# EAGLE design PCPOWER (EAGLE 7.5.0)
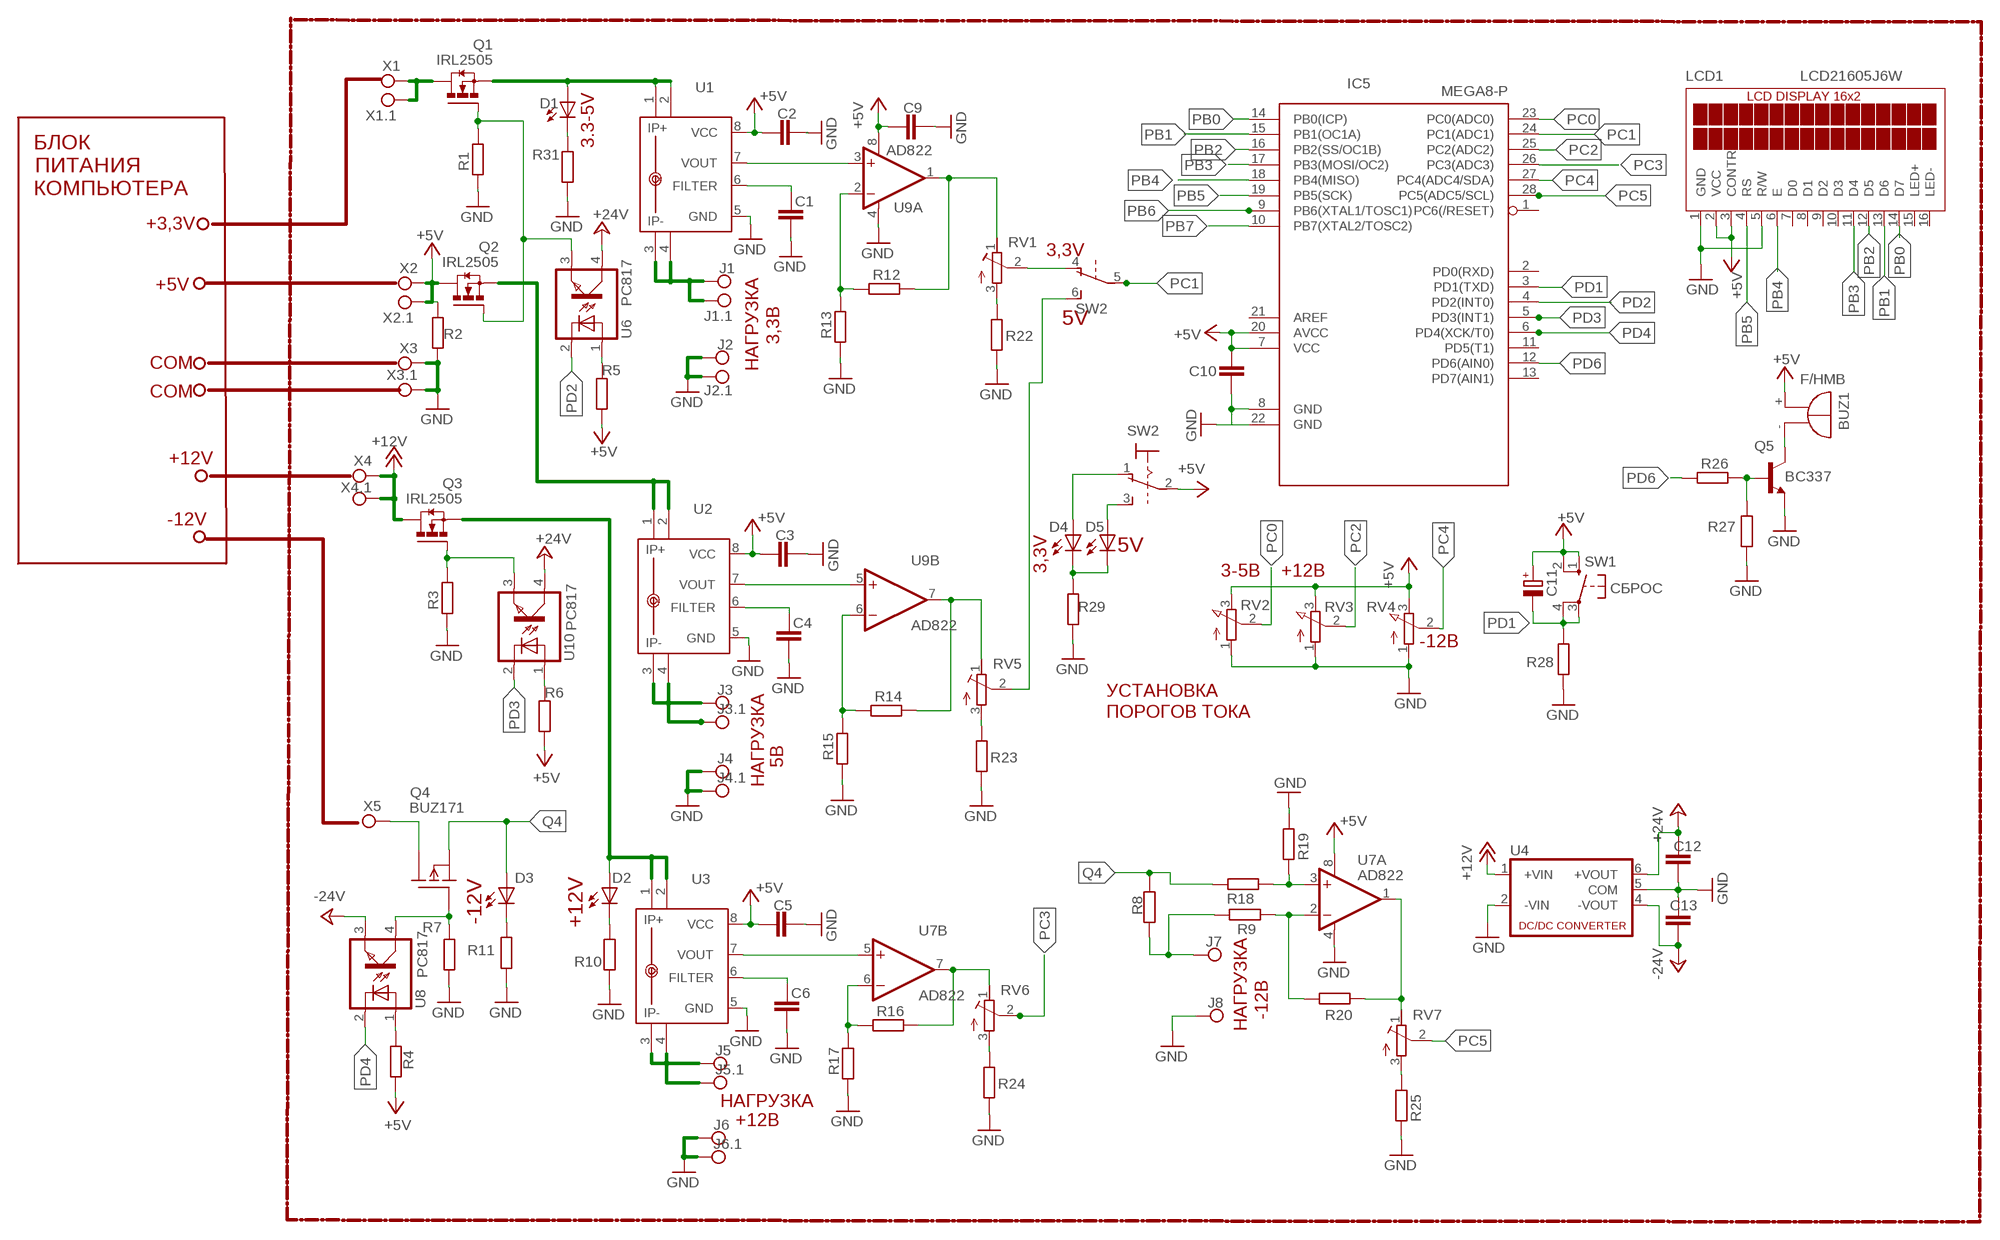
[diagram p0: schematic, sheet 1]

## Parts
BUZ1  F/HMB  [F/HMB]
C1  C-EUC1206  [C1206]
C2  C-EUC1206  [C1206]
C3  C-EUC1206  [C1206]
C4  C-EUC1206  [C1206]
C5  C-EUC1206  [C1206]
C6  C-EUC1206  [C1206]
C9  C-EUC1206  [C1206]
C10  C-EUC1206  [C1206]
C11  CPOL-EUE2-4  [E2-4]
C12  C-EUC1206  [C1206]
C13  C-EUC1206  [C1206]
D1  LED3MM  [LED3MM]
D2  LED3MM  [LED3MM]
D3  LED3MM  [LED3MM]
D4  LED3MM  [LED3MM]
D5  LED3MM  [LED3MM]
IC5  MEGA8-P  [DIL28-3]
J1  TPPAD1-20  [P1-20]
J1.1  TPPAD1-20  [P1-20]
J2  TPPAD1-20  [P1-20]
J2.1  TPPAD1-20  [P1-20]
J3  TPPAD1-20  [P1-20]
J3.1  TPPAD1-20  [P1-20]
J4  TPPAD1-20  [P1-20]
J4.1  TPPAD1-20  [P1-20]
J5  TPPAD1-20  [P1-20]
J5.1  TPPAD1-20  [P1-20]
J6  TPPAD1-20  [P1-20]
J6.1  TPPAD1-20  [P1-20]
J7  TPPAD1-20  [P1-20]
J8  TPPAD1-20  [P1-20]
LCD1  LCD21605J6W  [LCD21605J6W]
Q1  IRL2505  IRF3704L-V  [TO262-V]
Q2  IRL2505  IRF3704L-V  [TO262-V]
Q3  IRL2505  IRF3704L-V  [TO262-V]
Q4  BUZ171  [TO220]
Q5  BC337  [TO92]
R1  R-EU_R1206  [R1206]
R2  R-EU_VTA54  [VTA54]
R3  R-EU_R1206  [R1206]
R4  R-EU_R1206  [R1206]
R5  R-EU_R1206  [R1206]
R6  R-EU_R1206  [R1206]
R7  R-EU_R1206  [R1206]
R8  R-EU_0309/12  [0309/12]
R9  R-EU_R1206  [R1206]
R10  R-EU_R1206  [R1206]
R11  R-EU_R1206  [R1206]
R12  R-EU_R1206  [R1206]
R13  R-EU_R1206  [R1206]
R14  R-EU_R1206  [R1206]
R15  R-EU_R1206  [R1206]
R16  R-EU_R1206  [R1206]
R17  R-EU_R1206  [R1206]
R18  R-EU_R1206  [R1206]
R19  R-EU_R1206  [R1206]
R20  R-EU_R1206  [R1206]
R22  R-EU_R1206  [R1206]
R23  R-EU_R1206  [R1206]
R24  R-EU_R1206  [R1206]
R25  R-EU_R1206  [R1206]
R26  R-EU_R1206  [R1206]
R27  R-EU_R1206  [R1206]
R28  R-EU_R1206  [R1206]
R29  R-EU_R1206  [R1206]
R31  R-EU_R1206  [R1206]
RV1  R-TRIMM-3386-F  [R-TRIMM-3386F]
RV2  PTV09A  PV09A  [PTV09]
RV3  PTV09A  PV09A  [PTV09]
RV4  PTV09A  PV09A  [PTV09]
RV5  R-TRIMM-3386-F  [R-TRIMM-3386F]
RV6  R-TRIMM-3386-F  [R-TRIMM-3386F]
RV7  R-TRIMM-3386-F  [R-TRIMM-3386F]
SW1  SPST Push Button  10-XX  [B3F-10XX]
SW2  320-938  [320-938]
U1  ACS712ELCTR-20A-T  [SO8]
U2  ACS712ELCTR-20A-T  [SO8]
U3  ACS712ELCTR-20A-T  [SO8]
U4  NMA  [NMA]
U6  PC817  [DIL04]
U7  AD822  OPA2134P  [DIL08]
U8  PC817  [DIL04]
U9  AD822  OPA2134P  [DIL08]
U10  PC817  [DIL04]
X1  TPPAD1-20  [P1-20]
X1.1  TPPAD1-20  [P1-20]
X2  TPPAD1-20  [P1-20]
X2.1  TPPAD1-20  [P1-20]
X3  TPPAD1-20  [P1-20]
X3.1  TPPAD1-20  [P1-20]
X4  TPPAD1-20  [P1-20]
X4.1  TPPAD1-20  [P1-20]
X5  TPPAD1-20  [P1-20]

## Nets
+5V: BUZ1.+ C2.2 C3.2 C5.2 C9.2 C10.2 C11.+ IC5.7(VCC) IC5.20(AVCC) LCD1.2(VCC) LCD1.3(CONTR) Q2.2(D) R2.2 R4.2 R5.2 R6.2 RV2.3(E) RV3.3(E) RV4.3(E) SW1.1(S) SW1.2(S1) SW2.2(1:P) U1.8(VCC) U2.8(VCC) U3.8(VCC) U7.8(A:V+) U9.8(A:V+) X2.1.TP X2.TP
+12V: Q3.2(D) U4.1(+VIN) X4.1.TP X4.TP
+24V: C12.1 U4.6(+VOUT) U6.4(COL) U10.4(COL)
-24V: C13.2 U4.4(-VOUT) U8.3(EMIT)
GND: C1.2 C2.1 C3.1 C4.2 C5.1 C6.2 C9.1 C10.1 C12.2 C13.1 IC5.8(GND) IC5.22(GND) J2.1.TP J2.TP J4.1.TP J4.TP J6.1.TP J6.TP J8.TP LCD1.1(GND) LCD1.5(R/W) Q5.1(E) R1.2 R2.1 R3.2 R7.2 R10.2 R11.2 R13.2 R15.2 R17.2 R19.2 R22.2 R23.2 R24.2 R25.1 R27.2 R28.2 R29.2 R31.2 RV2.1(A) RV3.1(A) RV4.1(A) U1.5(GND) U2.5(GND) U3.5(GND) U4.2(-VIN) U4.5(COM) U7.4(A:V-) U9.4(A:V-) X3.1.TP X3.TP
N$1: R14.2 R15.1 U9.6(B:-IN)
N$2: J1.1.TP J1.TP U1.3(IP-) U1.4(IP-1)
N$3: R22.1 RV1.3(E)
N$4: Q5.2(B) R26.1 R27.1
N$5: D1.K(C) R31.1
N$6: BUZ1.- Q5.3(C)
N$7: RV1.2(S) SW2.4(B:O)
N$8: R14.1 RV5.1(A) U9.7(B:OUT)
N$9: R12.2 R13.1 U9.2(A:-IN)
N$10: R12.1 RV1.1(A) U9.1(A:OUT)
N$11: C1.1 U1.6(FILTER)
N$12: D1.A Q1.3(S) U1.1(IP+) U1.2(IP+1)
N$13: Q1.1(G) Q2.1(G) R1.1 U6.3(EMIT)
N$14: U1.7(VOUT) U9.3(A:+IN)
N$15: Q1.2(D) X1.1.TP X1.TP
N$16: R5.1 U6.1(A)
N$17: U2.7(VOUT) U9.5(B:+IN)
N$18: C4.1 U2.6(FILTER)
N$19: Q2.3(S) U2.1(IP+) U2.2(IP+1)
N$20: R23.1 RV5.3(E)
N$21: J3.1.TP J3.TP U2.3(IP-) U2.4(IP-1)
N$22: R16.2 R17.1 U7.6(B:-IN)
N$24: Q3.1(G) R3.1 U10.3(EMIT)
N$25: U3.7(VOUT) U7.5(B:+IN)
N$26: C6.1 U3.6(FILTER)
N$27: J5.1.TP J5.TP U3.3(IP-) U3.4(IP-1)
N$28: D2.K(C) R10.1
N$29: D2.A Q3.3(S) U3.1(IP+) U3.2(IP+1)
N$30: R16.1 RV6.1(A) U7.7(B:OUT)
N$31: R6.1 U10.1(A)
N$32: R24.1 RV6.3(E)
N$33: Q4.1(G) R7.1 U8.4(COL)
N$34: Q4.2(D) X5.TP
N$35: R4.1 U8.1(A)
N$36: D3.K(C) R11.1
N$37: J7.TP R8.1 R9.1
N$38: R9.2 R20.2 U7.2(A:-IN)
N$39: R18.2 R19.1 U7.3(A:+IN)
N$40: R20.1 RV7.1(A) U7.1(A:OUT)
N$41: R25.2 RV7.3(E)
N$42: D4.A SW2.1(1:O)
N$43: D5.A SW2.3(1:S)
N$44: D4.K(C) D5.K(C) R29.1
N$46: RV5.2(S) SW2.6(B:S)
PB0: IC5.14(PB0(ICP)) LCD1.14(D7)
PB1: IC5.15(PB1(OC1A)) LCD1.13(D6)
PB2: IC5.16(PB2(SS/OC1B)) LCD1.12(D5)
PB3: IC5.17(PB3(MOSI/OC2)) LCD1.11(D4)
PB4: IC5.18(PB4(MISO)) LCD1.6(E)
PB5: IC5.19(PB5(SCK)) LCD1.4(RS)
PB6: IC5.9(PB6(XTAL1/TOSC1))
PB7: IC5.10(PB7(XTAL2/TOSC2))
PC0: IC5.23(PC0(ADC0)) RV2.2(S)
PC1: IC5.24(PC1(ADC1)) SW2.5(B:P)
PC2: IC5.25(PC2(ADC2)) RV3.2(S)
PC3: IC5.26(PC3(ADC3)) RV6.2(S)
PC4: IC5.27(PC4(ADC4/SDA)) RV4.2(S)
PC5: IC5.28(PC5(ADC5/SCL)) RV7.2(S)
PD1: C11.- IC5.3(PD1(TXD)) R28.1 SW1.3(P) SW1.4(P1)
PD2: IC5.4(PD2(INT0)) U6.2(C)
PD3: IC5.5(PD3(INT1)) U10.2(C)
PD4: IC5.6(PD4(XCK/T0)) U8.2(C)
PD6: IC5.12(PD6(AIN0)) R26.2
Q4: D3.A Q4.3(S) R8.2 R18.1
Unconnected: IC5.1(PC6(/RESET)) IC5.2(PD0(RXD)) IC5.11(PD5(T1)) IC5.13(PD7(AIN1)) IC5.21(AREF) LCD1.7(D0) LCD1.8(D1) LCD1.9(D2) LCD1.10(D3) LCD1.15(LED+) LCD1.16(LED-)

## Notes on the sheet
- 3.3-5V
- БЛОК
- ПИТАНИЯ
- КОМПЬЮТЕРА
- +3,3V
- 3,3V
- +5V
- 5V
- 3,3В
- COM | НАГРУЗКА
- COM
- +12V
- -12V
- 5V
- 3-5В | +12В
- 3,3V
- СБРОС
- -12В
- УСТАНОВКА
- ПОРОГОВ ТОКА
- 5В
- НАГРУЗКА
- -12V | +12V
- -12В
- НАГРУЗКА
- НАГРУЗКА
- +12В

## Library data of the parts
BUZ1 = buzzer:F/HMB: BUZZER; OC_FARNELL: unknown; OC_NEWARK: unknown
C1-C6 C9 C10 C12 C13 = rcl:C-EU: CAPACITOR, European symbol
C11 = rcl:CPOL-EU: POLARIZED CAPACITOR, European symbol
D1-D5 = led:LED: LED
IC5 = atmel:MEGA8-P: MICROCONTROLLER 8 Kbytes FLASH, 1 kbytes SRAM, 512 bytes EEPROM, USART, 4-channel 10 bit ADC, 2-channel 8 bit ADC Pin compatible with Atmega48, ATMega88, ATMega168 Source: avr.lbr; OC_FARNELL: unknown; OC_NEWARK: unknown
J1 J1.1 J2 J2.1 J3 J3.1 J4 J4.1 J5 J5.1 J6 J6.1 J7 J8 X1 X1.1 X2 X2.1 X3 X3.1 X4 X4.1 X5 = testpad:TP: Test pad
LCD1 = display-lcd:LCD21605J6W
Q1-Q3 = transistor-power:IRF3704: SMPS MOSFET HEXFET® Power MOSFET Source: http://www.irf.com/product-info/datasheets/data/irf3704.pdf
Q4 = transistor-fet:BUZ171: P-Channel Enhancement MOSFET -50V; 7A; 0,4Ohm
Q5 = transistor:BC337: NPN TRANSISTOR
R1-R20 R22-R29 R31 = rcl:R-EU_: RESISTOR, European symbol
RV1 RV5-RV7 = rcl:R-TRIMM-3386-F
RV2-RV4 = pot:PV09A
SW1 = switch-omron:10-XX: OMRON SWITCH; MPN: B3F-1000; OC_FARNELL: 176432; OC_NEWARK: 36M3542
SW2 = switch:320-938: TOGGLE SWITCH distributor RS Components
U1-U3 = allegro:ACS712ELCTR-20A-T: Fully Integrated, Hall Effect-Based Linear Current Sensor with High Voltage Isolation and a Low-Resistance Current Conductor.
U4 = dc-dc-converter:NMA: DC-DC CONVERTER; MF: C & D TECHNOLOGIES, INC; MPN: NMA0515SC; OC_FARNELL: 1021434; OC_NEWARK: 61K3064
U6 U8 U10 = optocoupler:PC817: SHARP OPTO COUPLER; MPN: PC817X4J000F; OC_FARNELL: 9707727; OC_NEWARK: 97K7059
U7 U9 = burr-brown:OPA2134: Operational Amplifier; MF: TEXAS INSTRUMENTS; MPN: OPA2134PA; OC_FARNELL: 1097574; OC_NEWARK: 74K3897

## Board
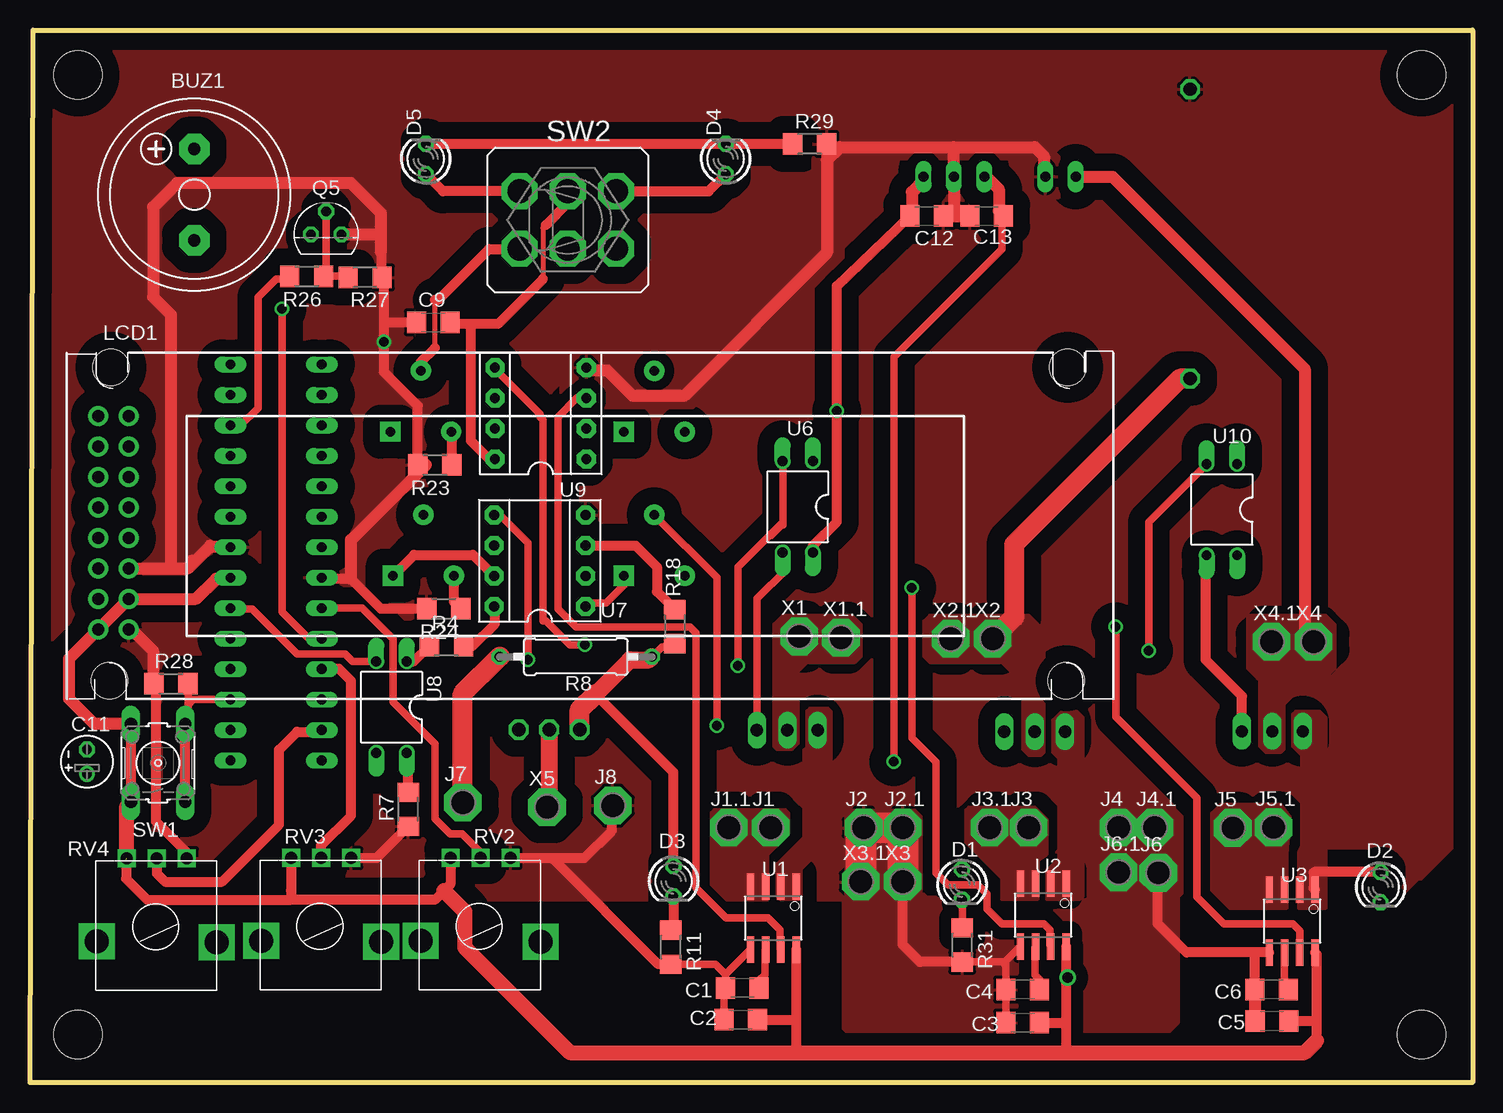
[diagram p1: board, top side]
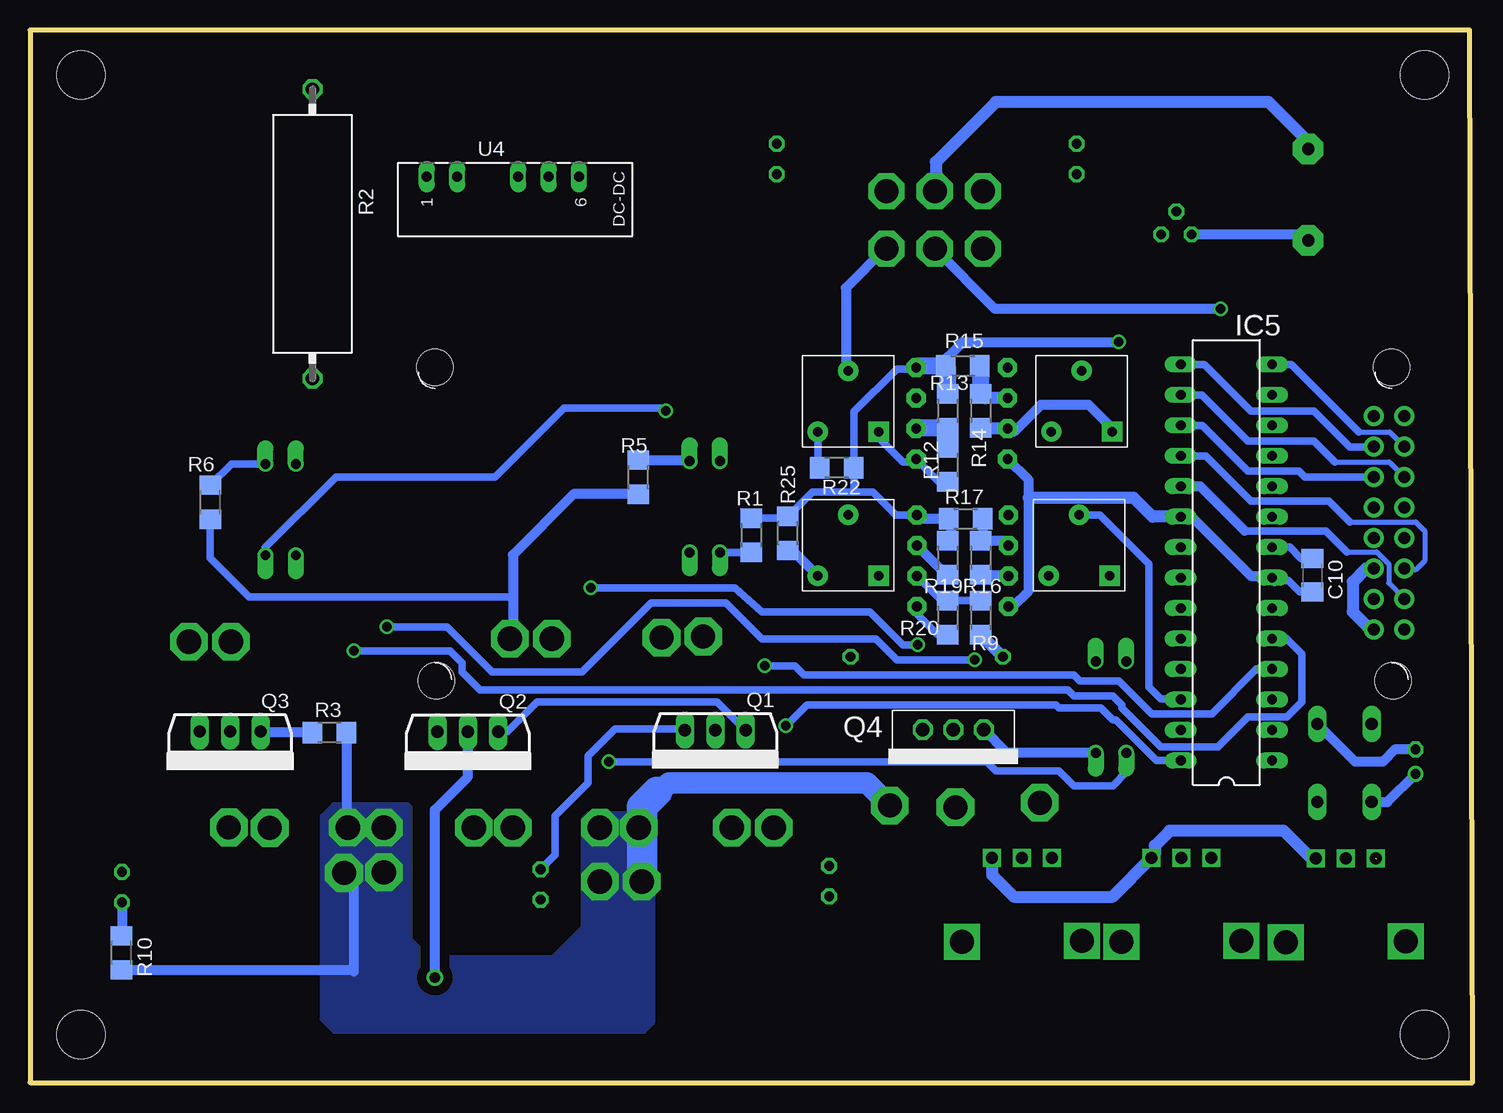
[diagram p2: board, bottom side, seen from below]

Size 120.25 x 87.75 mm. Coordinates in mm from the lower left corner, seen from the top.
Outline: 0,0 0.25,87.75 120.25,87.75 120.25,0 0,0
Copper layers (1*16): Top 0.035mm / dielectric 1.5mm / Bottom 0.035mm
Design rules "default *": minimum track width 10mil, minimum drill 24mil, track to track 5mil, track to pad 5mil, pad to pad 8mil, via to via 8mil, smd to smd 8mil, copper to edge 40mil, drill to drill 8mil, minimum pad ring 10mil, minimum via ring 8mil, stop-mask expansion 4mil, vias tented up to drill 0mil, thermal gap 10mil
Holes 4 mm at 4,84 4,4 116,4 116,84

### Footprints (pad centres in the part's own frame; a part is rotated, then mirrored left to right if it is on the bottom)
F/HMB = drill 1.016 pad 2.54 octagon: + 3.81,0; - -3.81,0
C1206 = smd 1.6 x 1.8: 1 -1.4,0; 2 1.4,0
E2-4 = drill 0.813 pad 1.27: + -1.016,0 | drill 0.813 pad 1.27 octagon: - 1.016,0
LED3MM = drill 0.813 octagon: A -1.27,0; K 1.27,0
DIL28-3 = drill 0.813 long: 1 -16.51,-3.81; 2 -13.97,-3.81; 3 -11.43,-3.81; 4 -8.89,-3.81; 5 -6.35,-3.81; 6 -3.81,-3.81; 7 -1.27,-3.81; 8 1.27,-3.81; 9 3.81,-3.81; 10 6.35,-3.81; 11 8.89,-3.81; 12 11.43,-3.81; 13 13.97,-3.81; 14 16.51,-3.81; 15 16.51,3.81; 16 13.97,3.81; 17 11.43,3.81; 18 8.89,3.81; 19 6.35,3.81; 20 3.81,3.81; 21 1.27,3.81; 22 -1.27,3.81; 23 -3.81,3.81; 24 -6.35,3.81; 25 -8.89,3.81; 26 -11.43,3.81; 27 -13.97,3.81; 28 -16.51,3.81
P1-20 = drill 2.007 pad 3.15 octagon: TP 0,0
LCD21605J6W = drill 1 pad 1.676: 1 2.47,-17.72; 2 -0.07,-17.72; 3 2.47,-15.18; 4 -0.07,-15.18; 5 2.47,-12.64; 6 -0.07,-12.64; 7 2.47,-10.1; 8 -0.07,-10.1; 9 2.47,-7.56; 10 -0.07,-7.56; 11 2.47,-5.02; 12 -0.07,-5.02; 13 2.47,-2.48; 14 -0.07,-2.48; 15 2.47,0.06; 16 -0.07,0.06 | hole 3: 0.875,-22; 1,4.125; 80.75,4.125; 80.625,-22
TO262-V = drill 1.016 long: 1 -2.54,0; 2 0,0; 3 2.54,0
TO220 = drill 1.118 octagon: 1 -2.54,0; 2 0,0; 3 2.54,0
TO92 = drill 0.813 octagon: 1 1.27,0; 2 0,1.905; 3 -1.27,0
R1206 = smd 1.6 x 1.803: 1 -1.422,0; 2 1.422,0
VTA54 = drill 1.1 octagon: 1 -12.065,0; 2 12.065,0
0309/12 = drill 0.813 octagon: 1 -6.35,0; 2 6.35,0
R-TRIMM-3386F = drill 0.8 pad 1.676 square: 1 0,0 | drill 0.8 pad 1.676: 2 5.08,2.54; 3 0,5.08
PTV09 = drill 1 square: 1 -2.5,0; 2 0,0; 3 2.5,0 | drill 2 square: P$4 -5,7; P$5 5,6.9
B3F-10XX = drill 1.016 long: 1 -3.251,2.261; 2 3.251,2.261; 3 -3.251,-2.261; 4 3.251,-2.261
320-938 = drill 2.007 octagon: 1 -2.388,4.013; 2 -2.388,0; 3 -2.388,-4.013; 4 2.388,4.013; 5 2.388,0; 6 2.388,-4.013
SO8 = smd 0.61 x 2.21: 1 0.635,-0.076; 2 1.905,-0.076; 3 3.175,-0.076; 4 4.445,-0.076; 5 4.445,5.156; 6 3.175,5.156; 7 1.905,5.156; 8 0.635,5.156
NMA = drill 0.813 long: 1 0,6.35; 2 0,3.81; 4 0,-1.27; 5 0,-3.81; 6 0,-6.35
DIL04 = drill 0.813 offset: 1 -1.27,-3.81; 2 1.27,-3.81; 3 1.27,3.81; 4 -1.27,3.81
DIL08 = drill 0.813 pad 1.6 octagon: 1 -3.81,-3.81; 2 -1.27,-3.81; 3 1.27,-3.81; 4 3.81,-3.81; 5 3.81,3.81; 6 1.27,3.81; 7 -1.27,3.81; 8 -3.81,3.81

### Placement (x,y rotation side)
BUZ1  13.7,74.02 90 top
C1  59.38,7.88 180 top
C2  59.25,5.25 0 top
C3  82.75,5 0 top
C4  82.75,7.75 180 top
C5  103.53,5.14 0 top
C6  103.5,7.75 180 top
C9  33.62,63.38 0 top
C10  13.36,42.29 270 bottom
C11  4.75,26.75 90 top
C12  74.75,72.25 0 top
C13  79.75,72.25 0 top
D1  77.69,16.51 270 top
D2  112.58,16.29 270 top
D3  53.63,16.79 270 top
D4  58,77 90 top
D5  33,77 90 top
IC5  20.51,43.36 90 bottom
J1  61.75,21.25 0 top
J1.1  58.25,21.25 0 top
J2  69.5,21.25 0 top
J2.1  72.75,21.25 0 top
J3  83.25,21.25 0 top
J3.1  80,21.25 0 top
J4  90.75,21.25 0 top
J4.1  93.75,21.25 0 top
J5  100.26,21.22 0 top
J5.1  103.67,21.27 0 top
J6  94.07,17.47 0 top
J6.1  90.75,17.52 0 top
J7  36.08,23.33 0 top
J8  48.58,23.09 0 top
LCD1  5.75,55.5 0 top
Q1  63.12,29.38 180 bottom
Q2  83.75,29.25 180 bottom
Q3  103.57,29.28 180 bottom
Q4  43.28,29.42 180 bottom
Q5  24.69,70.71 0 top
R1  60.12,45.62 90 bottom
R2  96.7,70.75 270 bottom
R3  95.29,29.17 0 bottom
R4  34.72,36.41 0 top
R5  69.53,50.47 270 bottom
R6  105.21,48.38 270 bottom
R7  31.54,22.77 270 top
R8  45.5,35.5 0 top
R9  41,38.75 90 bottom
R10  112.61,10.81 270 bottom
R11  53.42,11.29 270 top
R12  43.75,51.5 90 bottom
R13  43.75,56 90 bottom
R14  41,56 90 bottom
R15  42.5,59.75 180 bottom
R16  41,43.75 90 bottom
R17  42.25,47 180 bottom
R18  53.75,38 90 top
R19  43.75,43.75 90 bottom
R20  43.75,38.75 90 bottom
R22  53,51.25 0 bottom
R23  33.75,51.5 180 top
R24  34.5,39.5 180 top
R25  57.08,45.78 270 bottom
R26  23.06,67.21 180 top
R27  27.94,67.12 0 top
R28  11.75,33.25 180 top
R29  65,78.25 0 top
R31  77.71,11.47 270 top
RV1  49.5,54.25 90 bottom
RV2  37.55,18.72 180 top
RV3  24.27,18.72 180 top
RV4  10.57,18.69 180 top
RV5  30.04,54.26 90 bottom
RV6  30.25,42.25 90 bottom
RV7  49.5,42.25 90 bottom
SW1  10.67,26.64 90 top
SW2  44.83,71.91 270 top
U1  64.5,16.25 180 top
U2  87,16.5 180 top
U3  107.75,16 180 top
U4  80.83,75.52 90 bottom
U6  64,48 180 top
U7  42.5,43.5 90 top
U8  30.13,31.3 180 top
U9  42.57,55.79 90 top
U10  99.36,47.76 180 top
X1  64.13,37.19 0 top
X1.1  67.61,37.09 0 top
X2  80.25,37 0 top
X2.1  76.75,37 0 top
X3  72.75,16.75 0 top
X3.1  69.25,16.75 0 top
X4  107,36.75 0 top
X4.1  103.5,36.75 0 top
X5  43.1,22.95 0 top

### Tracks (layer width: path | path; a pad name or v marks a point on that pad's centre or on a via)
+5V  (via drill 0.9)  (1 unrouted)
  Top 0.406: 43,71.5 42.75,71.25 42.75,67
  Top 0.813: RV2.3 35.05,16.55 34.5,16 33.75,15.25 21.75,15.25 | 107.25,3.5 107.25,5 | 107.25,5 107.25,10.71 U3.8 | C5.2 107.11,5.14 107.25,5 | 86.36,5 U2.8 86.36,8.88 v86.5,8.75 | 86.36,5 86.36,2.63 86.5,2.5 | C3.2 86.36,5 | U1.8 63.87,5 | 63.87,5 63.87,2.62 63.75,2.5 | C2.2 63.62,5.25 63.87,5 | R4.2 36.91,36.41 38.75,38.25 38.75,39.63 U7.8 38.56,39.69 | SW1.2 SW1.1 | 8,18.62 8,17 9.75,15.25 21.75,15.25 | RV3.3 21.77,15.98 21.75,15.25 | U9.8 38.27,51.98 36.75,53.5 36.75,63.25 | 36.75,63.25 35.15,63.25 C9.2 | SW2.2 44.83,73.33 43,71.5 | 42.75,67 39,63.25 36.75,63.25
  Top 1.016: SW1.2 5.36,29.89 3.25,32 3.25,35.35 LCD1.2 LCD1.3 13.82,40.32 15.5,42 16.61,42 IC5.7
  Top 1.27: 107.25,3.5 106.25,2.5 86.5,2.5 63.75,2.5 45,2.5 36.25,11.25 36.25,14.25 34.5,16 | RV4.3 8.07,23.05 SW1.1
  Top 1.676: R2.2 95.86,58.69 82.03,44.85 82.03,38.77 X2.TP
  Bottom 0.61: R6.2 105.21,43.71 102,40.5 80.25,40.5 80,40.25 | C10.2 14.39,40.89 15.38,41.88 16.48,41.88 IC5.7
  Bottom 0.813: U7.8 38.31,39.69 37,41 37,48.75 37,50.22 U9.8 | R5.2 74.95,49.05 80,44 80,40.25 80,37.25 X2.TP | SW1.1 7.09,23.39 C11.+ | IC5.20 23.42,47.17 18.5,42.25 16.86,42.25 IC5.7 | v86.5,8.75 86.5,22.75 83.75,25.5 Q2.2
  Bottom 1.016: IC5.20 26.67,47.17 28.25,48.75 37,48.75 | 16.5,41.89 IC5.7 | BUZ1.+ 13.7,78.45 17,81.75 39.75,81.75 44.75,76.75 44.75,74.38 SW2.2
  pour Top (no thermals): 75,39 83.25,39 84.5,37.75 84.5,27.5 84.25,27.25 83.25,27.25 82.75,27.75 82.75,33.25 81,35 75,35 74.5,35.5 74.5,38.5
+12V
  Top 1.016: U4.1 90.23,75.52 106.25,59.5 106.25,36.5 X4.TP
  pour Top (no thermals): 102.5,28 102.5,33.5 101.5,34.5 101.5,39 108,39 108.75,38.25 108.75,34.5 107.75,33.5 106.5,33.5 104.5,31.5 104.5,27.75 104.25,27.5 103,27.5
+24V  (via drill 0.8)
  Top 0.813: U6.4 65.27,44.77 67.25,46.75 v67.25,56 67.25,66.4 C12.1
  Top 1.016: U4.6 74.48,75.23 73.5,74.25 73.5,72.4 C12.1
  Bottom 0.61: U10.4 100.63,44.62 94.75,50.5 81.5,50.5 75.75,56.25 67.5,56.25 v67.25,56
-24V  (via drill 0.8)
  Top 0.61: v72,26.75 72,60.5 81,69.5 81,72.1 C13.2
  Top 1.016: U4.4 79.73,75.52 80.75,74.5 80.75,72.65 C13.2
  Bottom 0.61: U8.3 28.86,25.89 30,24.75 33.25,24.75 34.5,26 39.75,26 40.5,26.75 v72,26.75
GND  (via drill 0.8)
  Top 0.61: C3.1 C4.2 81.35,9.75 | 81.35,9.75 81.35,10.14 U2.5 | R31.2 81.05,10.05 81.35,9.75 | C2.1 57.85,7.75 C1.2 57.98,9.01 | 57.98,9.01 U1.5 | R11.2 57.13,9.86 57.98,9.01
  Top 0.813: R24.2 29.25,39.5 26.75,42 24.41,42 IC5.22 | R23.2 32.33,56.42 29.5,59.25 v29.5,61.75 29.5,63.25 | 29.5,63.25 29.5,66.98 R27.2 29.25,67.23 29.25,69.25 | RV3.1 28.9,18.72 R7.2 | RV2.1 43.5,18.72 | 43.5,18.72 46.22,18.72 48.5,21 48.5,23.01 J8.TP | RV4.1 13.07,19.18 10.5,21.75 10.5,33.08 R28.2 | R11.2 52.36,9.86 43.5,18.72 | U3.5 102,10.84 | 102,10.84 96.41,10.84 94,13.25 94,17.4 J6.TP | C6.2 102.1,10.74 102,10.84 | C9.1 29.62,63.38 29.5,63.25 | R31.2 74.2,10.05 72.75,11.5 X3.TP
  Top 1.016: 26.75,42 26.75,45.25 33,51.5 R23.2 | LCD1.5 11.5,42.86 | 11.5,42.86 13.17,42.86 15,44.69 16.64,44.69 IC5.8 15.12,44.63 15,44.75 13.5,43.25 13.5,43.5 | LCD1.1 8.47,37.78 10.25,36 10.25,33.33 R28.2 | 77,78 67.5,78 66.42,76.92 R29.2 66.42,69.17 54.5,57.25 50.25,57.25 48.12,59.38 46.6,59.38 U9.4 | 77,78 83.75,78 84.5,77.25 84.5,75.66 U4.2 | 77,78 77.02,77.98 U4.5 77.02,72.48 77.25,72.25 | C12.2 77.25,72.25 | 77.25,72.25 C13.1 | 11.5,42.86 11.75,43.11 11.75,64 10.25,65.5 10.25,73 12.25,75 26.75,75 29.25,72.5 29.25,70.5 | 29.25,69.25 29.25,70.5 | Q5.1 29.04,70.71 29.25,70.5 | C6.2 102.1,5.17 C5.1
  Top 2.54: X3.TP J2.1.TP J2.TP 69.25,21 X3.1.TP
  Bottom 0.61: R1.2 57.23,47.05 R25.1 55.03,49.25 51.75,49.25 | U7.4 48.06,47.31 50,49.25 51.75,49.25 | 51.75,49.25 51.58,49.42 R22.2 51.58,55.92 48,59.5 46.48,59.5 U9.4 | C10.1 14.31,43.69 15.25,44.63 IC5.8
  Bottom 0.813: R19.2 43.5,45.42 43.5,46.75 43.67,46.92 R17.2 46,47 U7.4 | R13.2 43.75,60.5 42.5,61.75 v29.5,61.75 | R3.2 93.87,21.37 J4.1.TP | R10.2 93.39,9.39 93.25,9.25 93.25,16.65 J6.TP
  Bottom 1.016: 16.64,44.69 IC5.8 | LCD1.5 8.89,42.86 10,41.75 10,39.25 8.75,38 8.44,38 LCD1.1 | RV2.1 40.05,17.3 38.25,15.5 29.99,15.5 RV3.1 26.5,18.99 26.5,19.75 25.25,21 15.75,21 13.44,18.69 RV4.1
  Bottom 1.422: U9.4 46.23,59.75 R15.2 43.75,59.58 R13.2
  Bottom 1.778: 68,24.25 67.75,24.25 67,25 50.49,25 J8.TP
  Bottom 2.54: X3.1.TP 69.25,23 68,24.25
  pour Top (no thermals): 88.75,23 95.25,23 95.75,22.5 96,22.25 96,15.75 95.5,15.25 89.25,15.25 88.75,15.75 88.75,22.75
  pour Bottom (isolate 0.813, no thermals): 88.75,23.25 95,23.25 96,22.25 96,5.25 95,4.25 69,4.25 68.25,5 68.25,22 68.75,22.5 73.75,22.5 74.25,22 74.25,13 76.75,10.5 87,10.5 88.5,12 88.5,23
  pour Top (no thermals): 68,22.75 73.75,22.75 74.25,22.25 74.25,15.25 74,15 68.5,15 68,15.5
  pour Top (isolate 0.813): 45.25,61.75 57.25,61.75 61.75,66.25 65.25,69.75 65.25,79 66,79.75 83.25,79.75 85.75,77.25 85.75,73.75 84,73.75 83.5,74.25 83.5,76.75 83.25,77 69,77 67.75,75.75 67.75,68.75 55.25,56.25 45,56.25 44.25,57 44.25,61 45,61.75
  pour Top (isolate 1.422): 74.75,15 113.75,15 115.75,17 116,17 119.25,20.25 119.25,86.75 1.25,86.75 1.25,15.5 1.5,15.25 74.5,15.25
  pour Top (isolate 1.016): 67.75,23.25 67.75,4.5 68.25,4 94.75,4 95.75,5 95.75,22.5 95,23.25 88.75,23.25 88.5,23 88.5,15.75 88,15.25 74.75,15.5 73.75,16.5 74.25,22.25 73.25,23.25
N$1
  Bottom 1.016: U9.6 40.64,57.06 R14.2
  Bottom 1.422: R14.2 41,59.67 R15.1
N$2
  pour Top (no thermals): 61.5,15.25 61.5,19 63.25,20.75 63.25,22.5 63,22.75 57,22.75 56.75,22.5 56.75,16.5 58,15.25
N$3
  Bottom 0.61: RV1.3 54.58,51.16 R22.1
N$4
  Top 0.61: R27.1 26.43,67.21 R26.1 24.69,67.42 Q5.2
  Top 0.813: 26.39,67.25 R27.1
N$5
  Top 0.61: R31.1 77.71,15.22 D1.K
N$6
  Bottom 0.813: Q5.3 14.2,70.71 BUZ1.-
N$7
  Bottom 0.813: SW2.4 48.98,69.52 52.25,66.25 52.25,59.54 RV1.2
N$8
  Bottom 0.813: RV5.1 30.04,54.54 32,56.5 36,56.5 38.25,54.25 38.49,54.25 U9.7
  Bottom 1.016: R14.1 38.82,54.58 U9.7
N$9
  Bottom 1.422: R12.2 R13.1 46.32,54.58 U9.2
N$10
  Bottom 0.61: R12.1 44.48,50.08 U9.1 46.61,51.75 47.5,51.75 49.5,53.75 RV1.1
N$11
  Top 0.61: C1.1 60.77,8.53 61.25,9 61.25,11.02 U1.6
N$12
  Bottom 0.61: Q1.3 65.79,29.5 71.5,29.5 73.75,27.25 73.75,25 76.5,22.25 76.5,18.97 D1.A
  pour Top (no thermals): 62.25,15.5 62.25,18.25 64.5,20.5 64.5,27.75 64.75,28 64.75,31 65,31.25 66.5,31.25 66.75,31 66.75,26.5 66.25,26 66.25,19.75 64.25,17.75 64.25,15.25 62.5,15.25
N$13
  Top 0.61: Q1.1 60.59,40.34 63,42.75 63,43.92 U6.3
  Bottom 0.61: R1.1 62.72,44.2 U6.3 | Q2.1 80.5,29.25 78,31.75 62.96,31.75 Q1.1
N$14
  Top 0.61: U9.3 45.56,57.06 44,55.5 44,39.5 45.5,38 55,38 55.5,37.5 55.5,16.25 58,13.75 61.5,13.75 62.5,12.75 62.5,11.19 U1.7
N$15
  pour Top (no thermals): 62,28 62,38.25 62.75,39 68.5,39 69.25,38.25 69.25,35.5 68.75,35 64.75,35 64,34.25 64,28.25 63.5,27.75 62.25,27.75
N$16
  Bottom 0.813: R5.1 65.35,51.89 U6.1
N$17  (via drill 0.8)
  Top 0.61: U9.5 38.76,59.49 42.5,55.75 42.5,55.5 42.75,55.25 42.75,38.5 43,38.5 45,36.5 v46.25,36.5 | v73.5,41.25 73.5,28.75 75.5,26.75 75.5,17.5 76.5,16.5 79,16.5 79.75,15.75 79.75,14.5 81,13.25 84.5,13.25 85,12.75 85,11.44 U2.7
  Bottom 0.61: v46.25,36.5 47.5,36.5 50.25,39.25 59.25,39.25 61.5,41.25 v73.5,41.25
N$18
  Top 0.61: C4.1 84.15,8.6 83.75,9 83.75,11.27 U2.6
N$19
  pour Top (no thermals): 84.75,15.25 84.75,17.75 85.75,18.75 85.75,27 85.25,27.5 85.25,30.25 86,31 87.25,31 87.75,30.5 87.75,15.5 87.5,15.25
N$20
  Top 0.813: R23.1 35.17,54.21 RV5.3
N$21
  pour Top (no thermals): 78.25,23 83.75,23 84.75,22 84.75,19 84,18.5 84,15.25 81,15.25 81,17 78,20 78,22.75
N$22
  Bottom 0.813: U7.6 39.09,45.17 R16.2 40.83,45.34 R17.1
N$24
  Top 0.813: Q3.1 101.03,32.22 98,35.25 98,43.86 U10.3
  Bottom 0.813: R3.1 100.92,29.17 Q3.1
N$25  (via drill 0.8)
  Top 0.61: U7.5 39.19,47.31 41.5,45 v41.5,35.25 | v90.5,38 90.5,30.5 97.25,23.75 97.25,15.5 99.5,13.25 105.25,13.25 105.84,12.65 U3.7
  Bottom 0.61: v41.5,35.25 48,35.25 49.75,37 59.25,37 62.25,40 68.5,40 74.25,34.25 81.75,34.25 85.5,38 v90.5,38
N$26
  Top 0.61: U3.6 104.58,8.07 C6.1
N$27
  pour Top (no thermals): 99.25,23.25 104.25,23.25 105,22.25 104.75,19 104.75,14.5 100,14.5 98.5,16 98.5,22.5
N$28
  Bottom 0.813: D2.K 112.58,12.26 R10.1
N$29
  Top 0.813: D2.A 107.06,17.55 107,17.5 107,16.19 U3.1
  pour Top (no thermals): 105.75,14.5 105.75,19.25 106,19.75 106,27.25 105.25,28 105.25,30.75 105.5,31 107.5,31 108,30.5 108,14.5
N$30
  Top 0.813: RV6.1 32,44 36.92,44 U7.7
  Bottom 0.813: R16.1 38.79,42.33 U7.7
N$31
  Bottom 0.61: U10.1 103.44,51.57 R6.1
N$32
  Top 0.813: RV6.3 35.33,40.09 R24.1
N$33
  Top 0.813: R7.1 31.54,27.35 U8.4
  Bottom 0.813: U8.4 38.8,27.48 Q4.1
N$34
  Top 1.422: Q4.2 43.28,23.13 X5.TP
N$35
  Top 0.813: U8.1 31.99,35.1 R4.1
N$36
  Top 0.813: D3.K 53.63,12.92 R11.1
N$37
  Top 1.676: J7.TP 36.08,32.43 R8.1
  Bottom 1.016: R9.1 40.98,37.33 R8.1
N$38
  Bottom 0.61: R9.2 R20.2 44.25,40.17 U7.2
N$39
  Top 0.813: U7.3 50.48,44.77 52.25,43 52.25,40.92 R18.2
  Bottom 0.813: R19.1 43.87,42.33 U7.3
N$40
  Top 0.61: RV7.1 49.5,41.5 48,40 46.62,40 U7.1
  Bottom 0.61: R20.1 44.58,37.33 46.25,39 46.25,39.63 U7.1
N$41
  Bottom 0.813: R25.2 56.69,44.36 RV7.3
N$42
  Top 0.813: SW2.1 56.57,74.3 D4.A
N$43
  Top 0.813: SW2.3 34.43,74.3 D5.A
N$44
  Top 0.813: D5.K D4.K 58.02,78.25 R29.1
N$46
  Top 0.406: 33.75,61.25 33.75,65.25
  Top 0.813: RV5.2 32.58,60.08 33.75,61.25 | 33.75,65.25 34,65.25 38.25,69.5 40.79,69.5 SW2.6
PB0
  Bottom 0.406: 9.5,54.25 6.91,54.25 LCD1.14
  Bottom 0.61: IC5.14 15.12,59.87 9.5,54.25
PB1
  Bottom 0.61: IC5.15 22.37,59.87 18.5,56 13.25,56 10.25,53 8.24,53 LCD1.13
PB2
  Bottom 0.406: 11.5,51.75 6.95,51.75 LCD1.12
  Bottom 0.61: IC5.16 22.58,57.33 18.75,53.5 13.25,53.5 11.5,51.75
PB3
  Bottom 0.61: IC5.17 22.54,54.79 18.75,51 14.5,51 13.98,50.48 LCD1.11
PB4
  Bottom 0.406: 10.25,46.75 4.75,46.75 4,46 4,43.5 4.75,42.75 5.57,42.75 LCD1.6
  Bottom 0.61: IC5.18 22.25,52.25 18.5,48.5 12,48.5 10.25,46.75
PB5
  Bottom 0.406: 10.5,44.25 8,44.25 7,43.25 7,41.64 LCD1.4
  Bottom 0.61: 19,46 12.25,46 10.5,44.25
  Bottom 0.813: IC5.19 22.71,49.71 19,46
PC0
  Top 0.61: IC5.23 27.7,39.55 30.25,37 30.25,31.75 33.75,28.25 33.75,22 35,20.75 36,20.75 37.5,19.25 37.5,18.77 RV2.2
PC1  (via drill 0.8)
  Top 0.61: IC5.24 23.24,37.01 21,39.25 v21,64.5
  Bottom 0.813: SW2.5 39.81,64.5 v21,64.5
PC2
  Top 0.813: RV3.2 24.27,19.77 26.75,22.25 26.75,33.5 25.75,34.5 24.35,34.5 IC5.25
PC3
  Bottom 0.61: RV6.2 31.08,47.33 27,43.25 27,33 26,32 24.39,32 IC5.26
PC4
  Top 0.813: IC5.27 24.18,29.25 22.25,29.25 20.75,27.75 20.75,21.5 16,16.75 11.25,16.75 10.57,17.43 RV4.2
PC5  (via drill 0.8)
  Top 0.61: v57.25,29.75 57.25,42.12 RV7.2
  Bottom 0.61: IC5.28 26.35,26.85 29.75,30.25 30,30.25 31,31.25 34.5,31.25 34.75,31.5 55.5,31.5 v57.25,29.75
PD1
  Top 0.61: R28.1 13.17,31.5 | 13.17,31.5 13.17,30.13 SW1.4 | IC5.3 13.6,31.93 13.17,31.5
  Top 0.813: SW1.3 SW1.4
  Bottom 0.813: C11.- 6.48,27.77 7.5,26.75 9.79,26.75 SW1.4
PD2  (via drill 0.8)
  Top 0.406: 61.75,45.5 62.75,46.5
  Top 0.61: 62.75,46.5 62.75,46.75 | 62.75,46.75 62.75,51.79 U6.2 | v59,34.75 59,43 62.75,46.75
  Bottom 0.61: IC5.4 18.03,34.47 21.75,30.75 26.75,30.75 29.5,33.5 32.75,33.5 33.25,34 55.75,34 56.5,34.75 v59,34.75
PD3  (via drill 0.8)
  Top 0.61: v93.25,36 93.25,46.73 U10.2
  Bottom 0.61: IC5.5 15.51,37.01 14.25,35.75 14.25,31.75 15.5,30.5 18.75,30.5 21.25,28 26,28 29.25,31.25 29.25,31.5 30,32.25 33.25,32.25 33.75,32.75 82.75,32.75 84.25,34.25 84.25,35 85.25,36 v93.25,36
PD4
  Top 0.61: U8.2 26.89,35.1 26.25,35.75 22.25,35.75 18.5,39.5 16.75,39.5 IC5.6
PD6
  Top 0.61: IC5.12 17.54,54.79 19,56.25 19,65.5 20.5,67 21.43,67 R26.2
Q4
  Top 0.61: R18.1 52.68,36.33 R8.2
  Top 0.813: D3.A 53.63,25.86 47.12,32.38
  Top 1.422: 47.12,32.38 50,35.25 51.6,35.25 R8.2
  Top 1.676: Q4.3 45.82,31.07 47.12,32.38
